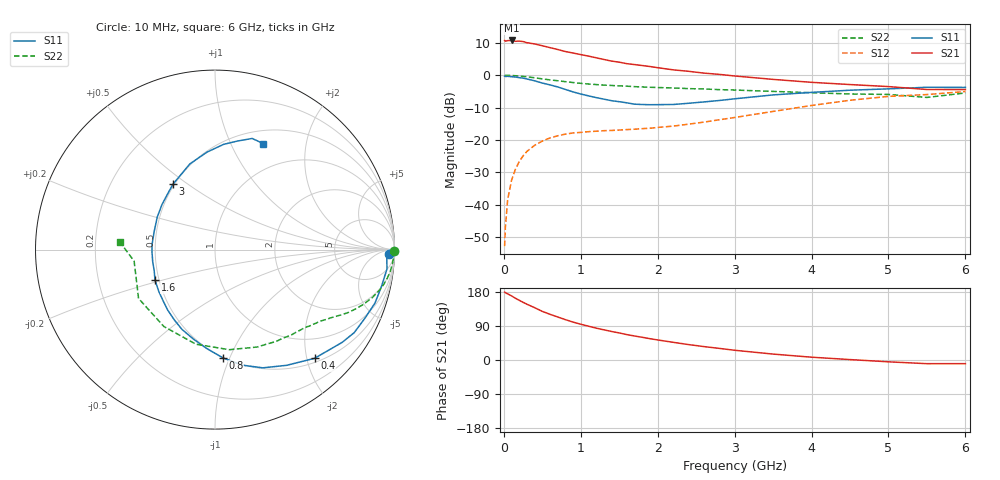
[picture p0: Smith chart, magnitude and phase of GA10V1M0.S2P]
! Infineon Technologies  Discrete & RF Semiconductors
! BF775
! Si NPN RF Bipolar Junction Transistor in SOT23
! VCE = 10 V  IC = 1 mA
! Common Emitter S-Parameters:  May  1996
# GHz  S  MA  R  50
!  f  S11  S21  S12  S22
! GHz  MAG  ANG  MAG  ANG  MAG  ANG  MAG  ANG
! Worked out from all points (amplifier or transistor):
!   36 points, 10 MHz to 6 GHz, reference 50 ohm
!   highest |S21| = 10.7 dB at 100 MHz (marker M1)
!   |S21| within 3 dB of that: start of sweep to 732.7 MHz
!   unconditionally stable (mu >= 1): 1.48 GHz to 3.391 GHz; 5.441 GHz to 5.649 GHz
!   at 250 MHz: K = 0.20, MSG = 17.7 dB, |S12| = -24.9 dB
!   at 1.4 GHz: K = 0.97, MSG = 10.7 dB, |S12| = -17.0 dB
!   at 6 GHz: K = 0.98, MSG = 0.3 dB, |S12| = -5.0 dB
!   S11 on the Smith chart (normalised r, x): 10 MHz: 41, -28; 400 MHz: 0.58, -2.14; 800 MHz: 0.50, -0.94; 1.6 GHz: 0.47, -0.19; 3 GHz: 0.49, +0.44; 6 GHz: 0.66, +1.34
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0.01  0.9676 -1.3  3.446 179.2  0.0023 90.8  0.9999 -0.4
0.02  0.9578 -2.4  3.358 177.6  0.0045 86.6  0.994 -1.0
0.05  0.9643 -6.4  3.429 174.5  0.0121 86.0  0.997 -2.4
0.1  0.95 -12.5  3.447 169.2  0.0239 81.7  0.9907 -4.8
0.15  0.9397 -18.5  3.347 163.0  0.0353 77.7  0.9838 -7.2
0.25  0.9032 -30.8  3.315 152.2  0.0569 70.9  0.9603 -11.6
0.4  0.8214 -47.5  3.046 138.1  0.083 61.9  0.9153 -17.1
0.5  0.7585 -58.2  2.858 128.3  0.0964 56.5  0.8796 -20.4
0.6  0.7105 -68.0  2.671 120.6  0.1077 51.9  0.8486 -23.0
0.8  0.6047 -85.8  2.324 106.5  0.1234 45.1  0.7967 -27.0
0.9  0.5534 -94.7  2.205 100.0  0.1287 42.9  0.7723 -28.7
1.1  0.4811 -112.5  1.976 89.2  0.1347 39.9  0.7333 -32.0
1.3  0.4279 -128.0  1.754 79.7  0.1395 38.4  0.7056 -34.6
1.6  0.3754 -152.9  1.509 67.0  0.145 38.4  0.6782 -38.8
1.9  0.3512 -177.0  1.364 56.2  0.1523 41.4  0.6534 -43.4
2.2  0.3538 163.0  1.213 46.7  0.164 44.2  0.6372 -48.5
3  0.4332 122.7  0.975 25.7  0.2229 50.1  0.5917 -66.5
3.5  0.4973 106.4  0.864 15.6  0.2766 49.2  0.5633 -81.9
4.5  0.588 85.4  0.719 1.1  0.4112 38.9  0.5145 -123.6
5  0.6172 78.4  0.669 -4.8  0.4723 30.6  0.5055 -147.4
5.5  0.653 71.5  0.603 -9.7  0.5038 20.7  0.4551 -171.9
6  0.6491 65.5  0.602 -9.6  0.561 15.6  0.5334 175.2
